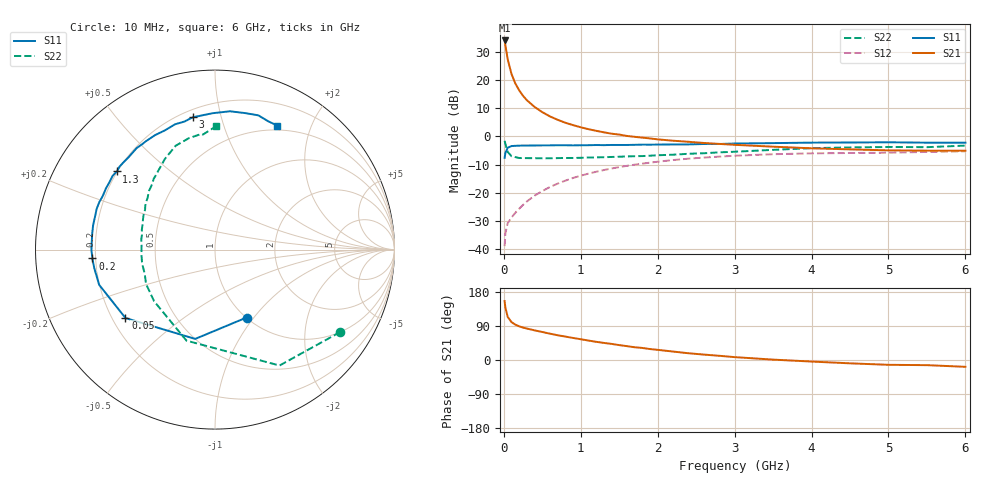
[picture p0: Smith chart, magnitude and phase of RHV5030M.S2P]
! SIEMENS Small Signal Semiconductors
! BFR106
! Si NPN RF Bipolar Junction Transistor in SOT23
! VCE = 0.5 V  IC = 30 mA
! Common Emitter S-Parameters:  August  1996
# GHz  S  MA  R  50
!  f  S11  S21  S12  S22
! GHz  MAG  ANG  MAG  ANG  MAG  ANG  MAG  ANG
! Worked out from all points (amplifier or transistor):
!   36 points, 10 MHz to 6 GHz, reference 50 ohm
!   highest |S21| = 34.0 dB at 10 MHz (marker M1)
!   |S21| within 3 dB of that: start of sweep to 28.12 MHz
!   unconditionally stable (mu >= 1): 227.6 MHz to end of sweep
!   at 250 MHz: K = 1.03, MAG = 18.3 dB, |S12| = -24.2 dB
!   at 1.4 GHz: K = 1.11, MAG = 4.1 dB, |S12| = -11.4 dB
!   at 6 GHz: K = 1.03, MAG = -1.0 dB, |S12| = -5.3 dB
!   S11 on the Smith chart (normalised r, x): 10 MHz: 1.00, -0.92; 50 MHz: 0.25, -0.32; 200 MHz: 0.19, -0.03; 1.3 GHz: 0.20, +0.34; 3 GHz: 0.24, +0.82; 6 GHz: 0.44, +1.53
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0.01  0.4173 -65.1  49.84 155.5  0.0114 71.3  0.835 -33.4
0.02  0.5097 -102.5  41.22 138.3  0.0192 58.4  0.7392 -60.9
0.05  0.6278 -142.6  23.2 113.8  0.0291 44.7  0.5315 -107.4
0.1  0.6746 -163.1  12.67 99.8  0.0367 46.6  0.4448 -139.7
0.15  0.6805 -171.2  8.585 93.2  0.0445 51.5  0.4293 -153.5
0.2  0.685 -175.9  6.519 88.9  0.0525 55.9  0.414 -161.1
0.25  0.6884 -179.8  5.203 85.5  0.0614 58.2  0.4128 -167.0
0.3  0.688 177.4  4.362 83.0  0.0706 60.6  0.4125 -170.4
0.4  0.69 172.5  3.315 78.2  0.0894 62.9  0.4108 -175.9
0.5  0.6926 168.6  2.682 73.9  0.1078 63.5  0.4097 180.0
0.6  0.6932 164.6  2.254 69.5  0.1272 63.4  0.4095 177.0
0.7  0.6973 161.0  1.964 65.3  0.146 62.6  0.4125 174.4
0.9  0.693 154.3  1.581 58.2  0.1838 60.0  0.4149 168.9
1.1  0.6978 147.5  1.341 51.3  0.2191 57.0  0.4223 164.9
1.3  0.6996 141.5  1.179 45.1  0.2537 53.4  0.4276 160.3
1.7  0.7089 130.3  0.982 33.6  0.3154 46.3  0.4457 152.3
2.2  0.7199 117.6  0.838 22.3  0.3809 36.9  0.4737 142.4
3  0.7474 99.5  0.709 7.6  0.4541 22.9  0.5349 127.2
3.5  0.76 91.0  0.657 1.0  0.4836 15.3  0.5774 118.9
4.5  0.7789 77.5  0.589 -8.8  0.5078 2.0  0.6373 103.3
5.5  0.7738 67.4  0.559 -13.6  0.5303 -5.7  0.6443 96.0
6  0.7734 63.3  0.558 -18.0  0.5445 -11.8  0.6865 89.6
